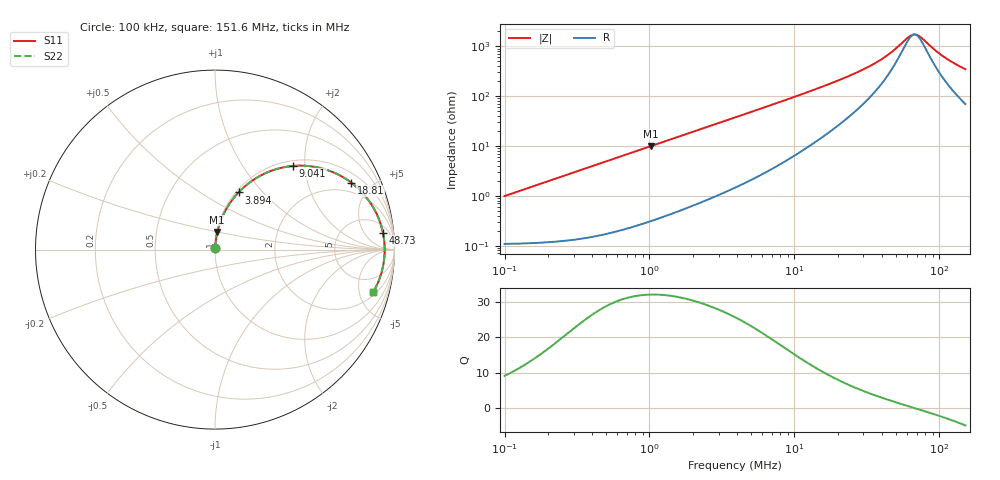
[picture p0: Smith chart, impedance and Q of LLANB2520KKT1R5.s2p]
! LLANB2520KKT1R5  S-PARAMETER MODEL  ( General Type )
! Model Generated by TAIYO YUDEN Corporation (http://www.ty-top.com)
! Version 1.0
! TAIYO YUDEN Control No. 160923NI42SB-FEC
! Copyright(c) 2016 TAIYO YUDEN CO.,LTD. All Rights Reserved.
! Product Description (link to TY-COMPAS)
! https://ds.yuden.co.jp/TYCOMPAS/or/detail?pn=LLANB2520KKT1R5M&u=M
! Products Name : Inductors
! Characteristics :
!  Inductance : 1.5 uH , SRF(min) : -Hz , DC Resistance(max) : 0.125 Ohm
!  Rated Current : Saturation :2300 mA , Temp Rise : 1800 mA (40 degC)
!  Case Size : 2.5 x 2.0 / 0.098 x 0.079 [mm/inch] , Thickness : 1 / 0.039 [mm/inch]
!  (Conditions: Temperature = 25 degC , DC Bias Current/Voltage = 0A / 0V)
! External Node Assignments :
!  1  o---GGG---o  2
! GND o---------o GND
! Frequency Range : 0.1MHz  -  151.640846MHz  [ 402 STEP ]
# MHz S RI R 50
! Freq[MHz].  S11 Real  S11 Imag  S21 Real  S21 Imag  S12 Real  S12 Imag  S22 Real  S22 Imag
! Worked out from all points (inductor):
!   401 points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, 100 kHz to 151.6 MHz, reference 50 ohm
!   read as one part in series: L = 1.56 uH near 103.7 kHz
!   highest Q = 32 at 1.023 MHz (marker M1), where L = 1.54 uH
!   self-resonance near 67.53 MHz
!   S11 on the Smith chart (normalised r, x): 100 kHz: 1.00, +0.02; 3.894 MHz: 1.03, +0.74; 9.041 MHz: 1.11, +1.74; 18.81 MHz: 1.45, +3.80; 48.73 MHz: 9, +15; 151.6 MHz: 2.39, -6.79
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0.1  0.00118 0.00979  0.9988 -0.00979  0.9988 -0.00979  0.00118 0.00979
0.341025  0.00249 0.0333  0.9975 -0.0333  0.9975 -0.0333  0.00249 0.0333
1.023079  0.0128 0.0977  0.9872 -0.0977  0.9872 -0.0977  0.0128 0.0977
1.162983  0.0159 0.1105  0.9841 -0.1105  0.9841 -0.1105  0.0159 0.1105
2.33212  0.0543 0.2102  0.9457 -0.2102  0.9457 -0.2102  0.0543 0.2102
3.894109  0.1312 0.3187  0.8688 -0.3187  0.8688 -0.3187  0.1312 0.3187
5.825765  0.2467 0.4085  0.7533 -0.4085  0.7533 -0.4085  0.2467 0.4085
9.040698  0.4347 0.4661  0.5653 -0.4661  0.5653 -0.4661  0.4347 0.4661
13.2799  0.619 0.4456  0.381 -0.4456  0.381 -0.4456  0.619 0.4456
18.80544  0.7601 0.3723  0.2399 -0.3723  0.2399 -0.3723  0.7601 0.3723
30.83107  0.8858 0.2277  0.1142 -0.2277  0.1142 -0.2277  0.8858 0.2277
37.7104  0.9142 0.1671  0.0858 -0.1671  0.0858 -0.1671  0.9142 0.1671
45.28783  0.9312 0.1134  0.0688 -0.1134  0.0688 -0.1134  0.9312 0.1134
48.72924  0.936 0.0923  0.064 -0.0923  0.064 -0.0923  0.936 0.0923
61.8253  0.9446 0.0248  0.0554 -0.0248  0.0554 -0.0248  0.9446 0.0248
65.31641  0.9452 0.00937  0.0548 -0.00937  0.0548 -0.00937  0.9452 0.00937
69.00467  0.9453 -0.00605  0.0547 0.00605  0.0547 0.00605  0.9453 -0.00605
75.62035  0.9443 -0.0318  0.0557 0.0318  0.0557 0.0318  0.9443 -0.0318
92.49348  0.9369 -0.089  0.0631 0.089  0.0631 0.089  0.9369 -0.089
107.0847  0.9268 -0.1314  0.0732 0.1314  0.0732 0.1314  0.9268 -0.1314
128.602  0.9074 -0.1858  0.0926 0.1858  0.0926 0.1858  0.9074 -0.1858
151.6408  0.8824 -0.2359  0.1176 0.2359  0.1176 0.2359  0.8824 -0.2359
